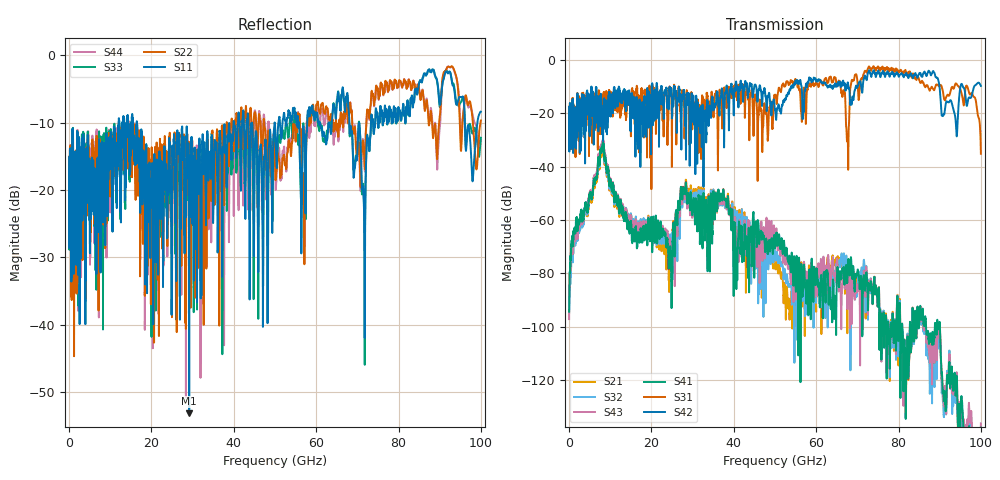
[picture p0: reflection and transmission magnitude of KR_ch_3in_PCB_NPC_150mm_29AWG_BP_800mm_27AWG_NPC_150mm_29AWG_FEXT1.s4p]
# GHz S RI R 45
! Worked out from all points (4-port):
!   4000 points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, 25 MHz to 100 GHz, reference 45 ohm
!   strongest paths, dB at 25 MHz, 25.02 GHz, 50.02 GHz, 75.03 GHz, 100 GHz:
!     S42: -22.2, -20.8, -18.7, -4.1, -9.8
!     S31: -22.1, -22.1, -13.3, -2.4, -35.2
!     S41: -94.3, -77.0, -70.6, -92.0, -137.7
!     S43: -97.1, -70.6, -70.5, -91.9, -136.1
!     S32: -94.6, -65.9, -72.6, -91.7, -142.1
!     S21: -88.6, -67.5, -76.4, -91.7, -142.8
!   lowest |S11| = -53.1 dB at 29.18 GHz (marker M1), VSWR 1.00, Z = 44.9 + j0.151 ohm
!   |S11| at or under -10 dB: start of sweep to 12.08 GHz; 16.48 GHz to 39.96 GHz (23.48 GHz wide, 83.2 % of centre); 43.53 GHz to 49.92 GHz (6.387 GHz wide, 13.7 % of centre)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
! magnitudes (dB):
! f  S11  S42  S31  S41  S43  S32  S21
! 25 MHz  -17.4  -22.2  -22.1  -94.3  -97.1  -94.6  -88.6
! 8.025 GHz  -15.7  -27.9  -17.6  -32.5  -30.9  -32.5  -34.0
! 24 GHz  -18.2  -15.9  -22.7  -68.9  -65.3  -66.2  -71.4
! 29.18 GHz  -53.1  -16.4  -31.7  -51.0  -53.0  -49.8  -48.6
! 67.62 GHz  -5.8  -8.7  -28.3  -80.5  -89.4  -87.3  -89.9
! 77.2 GHz  -9.6  -4.6  -2.7  -108.0  -107.4  -105.3  -107.3
! 100 GHz  -8.4  -9.8  -35.2  -137.7  -136.1  -142.1  -142.8
